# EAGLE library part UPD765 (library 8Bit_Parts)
µPD765 MFM Disk Controller
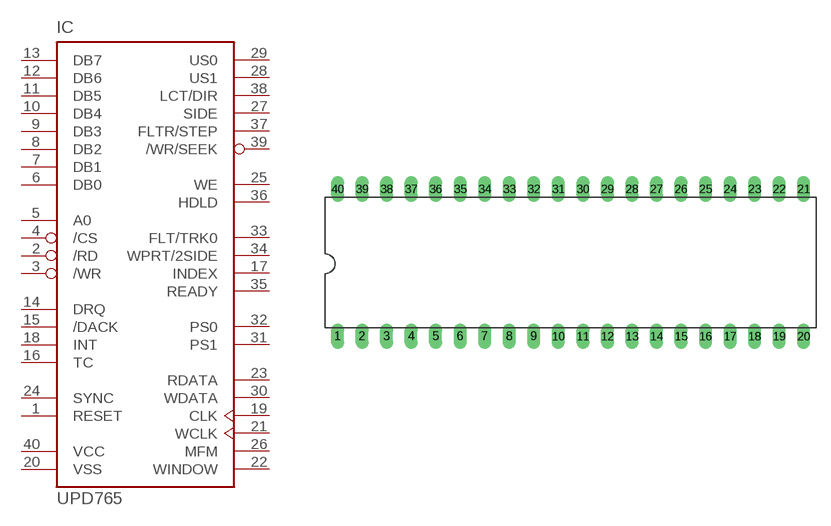
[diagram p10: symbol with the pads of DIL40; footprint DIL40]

Designator prefix IC

## UPD765  [DIL40]
1  RESET  in
2  /RD  in
3  /WR  in
4  /CS  in
5  A0  in
6  DB0
7  DB1
8  DB2
9  DB3
10  DB4
11  DB5
12  DB6
13  DB7
14  DRQ  out
15  /DACK  in
16  TC  in
17  INDEX  in
18  INT  out
19  CLK  in
20  VSS  pwr
21  WCLK  in
22  WINDOW  in
23  RDATA  in
24  SYNC  out
25  WE  out
26  MFM  out
27  SIDE  out
28  US1  out
29  US0  out
30  WDATA  out
31  PS1  out
32  PS0  out
33  FLT/TRK0  in
34  WPRT/2SIDE  in
35  READY  in
36  HDLD  out
37  FLTR/STEP  out
38  LCT/DIR  out
39  /WR/SEEK  out
40  VCC  pwr

## Footprint DIL40 (pad centres in mm)
Dual In Line Package
drill 0.813 long: 1 -24.13,-7.62; 2 -21.59,-7.62; 3 -19.05,-7.62; 4 -16.51,-7.62; 5 -13.97,-7.62; 6 -11.43,-7.62; 7 -8.89,-7.62; 8 -6.35,-7.62; 9 -3.81,-7.62; 10 -1.27,-7.62; 11 1.27,-7.62; 12 3.81,-7.62; 13 6.35,-7.62; 14 8.89,-7.62; 15 11.43,-7.62; 16 13.97,-7.62; 17 16.51,-7.62; 18 19.05,-7.62; 19 21.59,-7.62; 20 24.13,-7.62; 21 24.13,7.62; 22 21.59,7.62; 23 19.05,7.62; 24 16.51,7.62; 25 13.97,7.62; 26 11.43,7.62; 27 8.89,7.62; 28 6.35,7.62; 29 3.81,7.62; 30 1.27,7.62; 31 -1.27,7.62; 32 -3.81,7.62; 33 -6.35,7.62; 34 -8.89,7.62; 35 -11.43,7.62; 36 -13.97,7.62; 37 -16.51,7.62; 38 -19.05,7.62; 39 -21.59,7.62; 40 -24.13,7.62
